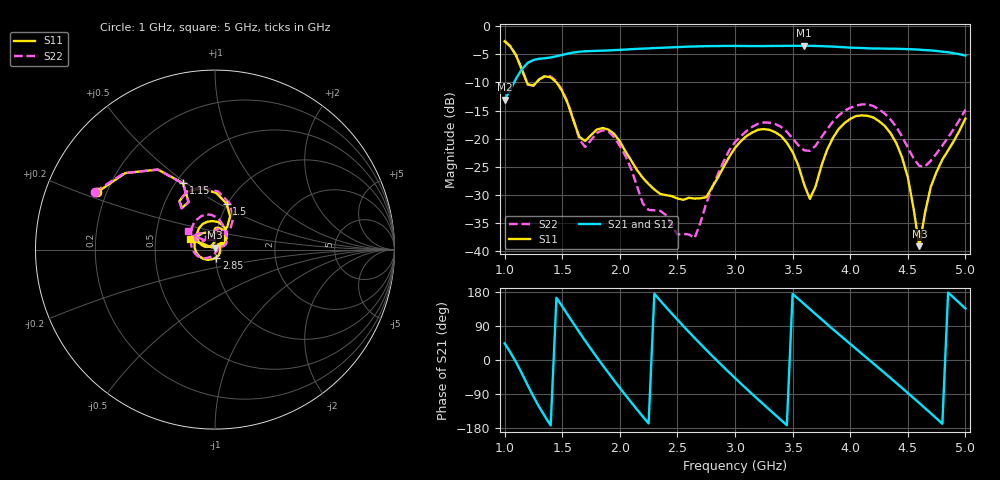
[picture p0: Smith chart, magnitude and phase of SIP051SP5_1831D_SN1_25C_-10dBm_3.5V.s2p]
# GHz  S  dB  R  50
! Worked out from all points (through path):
!   81 points, 1 GHz to 5 GHz, reference 50 ohm
!   highest |S21| = -3.52 dB at 3.6 GHz (marker M1); lowest = -13.1 dB at 1 GHz (marker M2)
!   lowest |S11| = -39.1 dB at 4.6 GHz (marker M3), VSWR 1.02, Z = 50 + j1.11 ohm
!   |S11| at or under -10 dB: 1.194 GHz to 1.276 GHz (82.61 MHz wide, 6.69 % of centre); 1.45 GHz to end of sweep
!   |S22| runs from -37.6 to -2.6 dB; largest |S21 - S12| = 0.0036
!   S11 on the Smith chart (normalised r, x): 1 GHz: 0.16, +0.22; 1.15 GHz: 0.55, +0.48; 1.5 GHz: 0.99, +0.55; 2.85 GHz: 1.01, -0.09; 5 GHz: 0.75, +0.09
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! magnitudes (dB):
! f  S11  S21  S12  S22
! 1 GHz  -2.7  -13.1  -13.1  -2.6
! 1.15 GHz  -7.7  -7.7  -7.7  -7.8
! 1.2 GHz  -10.3  -6.6  -6.6  -10.4
! 1.5 GHz  -11.6  -5.1  -5.1  -11.4
! 1.7 GHz  -20.4  -4.5  -4.5  -21.5
! 1.9 GHz  -18.4  -4.3  -4.3  -18.7
! 2.2 GHz  -27.0  -4.0  -4.0  -31.5
! 2.35 GHz  -29.8  -3.9  -3.9  -32.8
! 2.65 GHz  -30.6  -3.6  -3.6  -37.6
! 2.85 GHz  -26.9  -3.6  -3.6  -26.3
! 3 GHz  -21.6  -3.5  -3.5  -20.6
! 3.35 GHz  -18.9  -3.5  -3.6  -17.4
! 3.6 GHz  -28.1  -3.5  -3.5  -22.0
! 3.65 GHz  -30.7  -3.5  -3.5  -22.2
! 3.7 GHz  -28.4  -3.6  -3.6  -21.2
! 3.85 GHz  -19.9  -3.7  -3.7  -17.0
! 4 GHz  -16.5  -3.8  -3.8  -14.5
! 4.35 GHz  -19.0  -4.0  -4.0  -16.6
! 4.5 GHz  -26.8  -4.1  -4.1  -21.5
! 4.6 GHz  -39.1  -4.2  -4.2  -24.8
! 4.7 GHz  -28.5  -4.3  -4.3  -23.9
! 5 GHz  -16.4  -5.2  -5.3  -14.9
